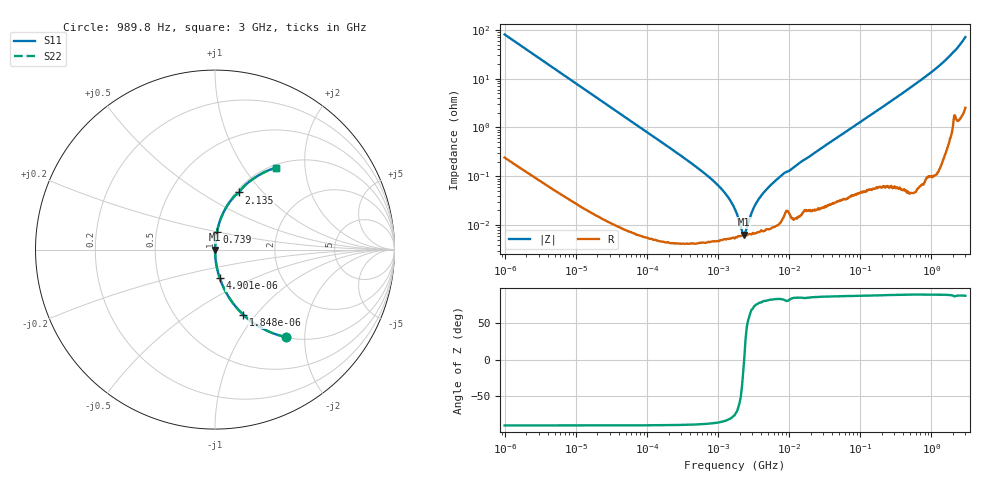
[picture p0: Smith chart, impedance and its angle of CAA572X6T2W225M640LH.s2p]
! S-Parameter Data Generated by TDK Corporation
! Copyright(C) 2024 TDK Corporation.
! All Rights Reserved.
! TDK P/N: CAA572X6T2W225M640LH (Multilayer Ceramic Chip Capacitor)
! Property: C=2.2uF
! Size(LxWxT): 6x5x6.4mm
! Model Type: s2p (Touchstone File Format Version 1.0)
! Frequency: DC=Yes Start=0.000989846MHz Stop=3000MHz 523points Log-sweep
! Model Generated on May 28, 2024
! Terms and conditions regarding TDK Simulation Models:
! 1)This simulation model is being provided solely for informational
!  purposes. Please refer to the specifications of the products in
!  terms of detailed characteristics of such products.
! 2)In no event shall TDK Corporation of any of its subsidiaries be
!  liable for any loss or damage arising, directly or indirectly,
!  from any information contained in this simulation model, including,
!  but not limited to loss or damages arising from any inaccuracies,
!  omissions or errors in connection with such information.
! 3)Any and all copyrights on this simulation model are owned by
!  TDK Corporation.  Duplication or redistribution of this simulation
!  model without prior written permission from TDK Corporation
!  is prohibited.
! 4)This simulation model is subject to any modification or change
!  without any prior notice.
! 5)Neither TDK Corporation nor any of its subsidiaries shall make any
!  warranty, express or implied, including but not limited to the
!  correctness, implied warranties of merchantability and fitness for
!  a particular purpose with respect to this simulation models.
! 6)The use of this simulation model shall be deemed to have consented
!  to the terms and conditions hereof.
! Port Assignments:
!  1 ---| |--- 2
! Applicable Conditions:
!  Temperature = 25 degC
!  DC Bias Voltage = 0 V
!  Small Signal Operation
# Hz S MA R 50
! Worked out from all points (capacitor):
!   522 points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, 989.8 Hz to 3 GHz, reference 50 ohm
!   read as one part in series: C = 2 uF near 1.07 kHz
!   lowest |Z| = 6.41 mohm at 2.332 MHz (marker M1)
!   series resonance near 2.317 MHz, so ESL is about 2.4 nH
!   S11 on the Smith chart (normalised r, x): 989.8 Hz: 1.00, -1.61; 1.848 kHz: 1.00, -0.86; 4.901 kHz: 1.00, -0.33; 739 MHz: 1.00, +0.20; 2.135 GHz: 1.04, +0.75; 3 GHz: 1.05, +1.42
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989.846  0.6259 -51.1  0.778 38.8  0.778 38.8  0.6259 -51.1
1847.96  0.3957 -66.5  0.9172 23.3  0.9172 23.3  0.3957 -66.5
4901.49  0.1608 -80.6  0.9865 9.3  0.9865 9.3  0.1608 -80.6
12024.6  0.06641 -86.0  0.9976 3.8  0.9976 3.8  0.06641 -86.0
146075  0.005481 -89.2  0.9999 0.3  0.9999 0.3  0.005481 -89.2
452889  0.001704 -88.5  1 0.1  1 0.1  0.001704 -88.5
879151  0.0007775 -86.5  1 0.0  1 0.0  0.0007775 -86.5
1350400  0.00039 -82.3  0.9999 0.0  0.9999 0.0  0.00039 -82.3
1774520  0.000191 -72.6  0.9999 0.0  0.9999 0.0  0.000191 -72.6
2074250  9.412e-05 -51.1  0.9999 0.0  0.9999 0.0  9.412e-05 -51.1
2331840  6.412e-05 3.5  0.9999 -0.0  0.9999 -0.0  6.412e-05 3.5
2621410  0.000108 53.2  0.9999 -0.0  0.9999 -0.0  0.000108 53.2
3186110  0.0002325 73.3  0.9999 -0.0  0.9999 -0.0  0.0002325 73.3
3581770  0.0003125 76.8  0.9999 -0.0  0.9999 -0.0  0.0003125 76.8
5088690  0.0005956 82.1  0.9999 -0.0  0.9999 -0.0  0.0005956 82.1
8127370  0.001106 82.8  0.9999 -0.1  0.9999 -0.1  0.001106 82.8
2.09559e7  0.002772 85.8  0.9998 -0.2  0.9998 -0.2  0.002772 85.8
2.50734e8  0.03219 87.1  0.9989 -1.8  0.9989 -1.8  0.03219 87.1
7.38967e8  0.0974 84.0  0.9946 -5.6  0.9946 -5.6  0.0974 84.0
1.45942e9  0.211 77.2  0.9754 -12.2  0.9754 -12.2  0.211 77.2
2.13473e9  0.3454 67.1  0.9222 -20.2  0.9222 -20.2  0.3454 67.1
3e9  0.5699 53.2  0.8017 -34.7  0.8017 -34.7  0.5699 53.2
